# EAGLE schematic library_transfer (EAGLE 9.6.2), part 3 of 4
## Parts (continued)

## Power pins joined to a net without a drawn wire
3V3(OUT): U73.36(3V3(OUT))
3V3OUT: U181.17(3V3OUT)
ADC_AVDD: U70.43(ADC_AVDD)
AGND: U181.25(AGND)
DVDD: U70.23(DVDD) U70.50(DVDD)
EXP: U38.29(EXP)
GND: U34.1(GND) U38.15(GND) U38.23(GND) U38.26(GND) U70.57(GND) U73.3(GND) U73.8(GND) U73.13(GND) U73.18(GND) U73.23(GND) U73.28(GND) U73.33(GND) U73.38(GND) U135.16(GND) U147.1(GND)
GND1: U181.7(GND1)
GND2: U181.18(GND2)
GND3: U181.21(GND3)
GND_2: U135.1(GND_2)
GND_3: U135.6(GND_3)
GND_4: U135.8(GND_4)
GND_5: U135.9(GND_5)
IOVDD: U70.1(IOVDD) U70.10(IOVDD) U70.22(IOVDD) U70.33(IOVDD) U70.42(IOVDD) U70.49(IOVDD)
SWGND: U73.42(SWGND)
USB_VDD: U70.48(USB_VDD)
V+: U34.8(V+) U147.8(V+)
VBAT_ANA: U38.3(VBAT_ANA)
VBAT_DIG: U38.14(VBAT_DIG)
VBAT_RF: U38.24(VBAT_RF)
VBUS: U73.40(VBUS)
VCC: U115.14(VCC) U181.20(VCC)
VCCIO: U181.4(VCCIO)
VR_ANA: U38.2(VR_ANA)
VR_DIG: U38.4(VR_DIG)
VR_PA: U38.25(VR_PA)
VSYS: U73.39(VSYS)

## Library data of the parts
A1 = ruark2:SA818: NiceRF SA818 1W Embedded walkie talkie module
A2 = ruark2:RFM69HCW: RFM69HCW WIRELESS TRANSCEIVER 91; PARTNO: 1568-1394-ND
A3 = ruark2:PCN2-S: Isolated Module DC DC Converter 1 Output 12V 167mA 10.8V - 13.2V Input; PARTNO: 102-3935-ND
A4 = ruark2:DGVVII: Gan Module Foolishness
ANT1 = ruark2:W3010: 2.8dBi Chip antenna 1.575GHz - Antennas ROHS; JLCPCB: C6926293
ANT2 = ruark2:ANT-916-HETH: RF ANT 916MHZ HELICAL SLD TH
ANT3 = ruark2:ANT-433-HETH: 433MHz Alarms, ISM, Remote Control, Security Systems Helical RF Antenna 418MHz ~ 458MHz 1.9dBi Solder Through Hole; PARTNO: ANT-433-HETH-ND
B1 = ruark2:LEAF_BATTERY_PN: Nissan Leaf Battery P, M, N
B2 = ruark2:LEAF_BATTERY_NP: Nissan Leaf Battery N, M, P
B3 = ruark2:BU-2032SM-JJ-G
B4 = ruark2:BK-18650-PC4: HOLDER BATT LI-ION 2CELL 4PC PIN; PARTNO: BK-18650-PC4-ND
B5 = ruark2:BK-912: HOLDER COIN CELL 20MM SMD CR2032 2032; PARTNO: BK-912-ND
B6 = ruark2:BH-18650-B1BA002: 18650 JLCPCB
B7 = ruark2:BH-123A-A5BJ002: Battery case CR123A - Button And Strip Battery Connector ROHS; JLCPCB: C5290177
B8 = ruark2:BH-102B-5: Battery Holder (Open) AAA 2 Cell SMD (SMT) Tab; PARTNO: 2057-BH-102B-5-ND
B9 = ruark2:AN-2852-A: PCB Outline for Flanged Box: Metal, Aluminum Natural Cover Included 4.530" L x 2.560" W (115.06mm x 65.02mm) X 1.180" (29.97mm); PARTNO: 377-2364-ND
B10 = ruark2:AN-1320-A: PCB Outline for: Box Metal, Aluminum Natural Cover Included 4.040" L x 2.070" W (102.62mm x 52.58mm) X 1.000" (25.40mm); PARTNO: 377-2405-ND
B11 B12 = ruark2:18350: Ecigarette Battery
B13 = ruark2:2479: HOLDER BATTERY 3CELL AAA PC MNT; PARTNO: 36-2479-ND
B14 = ruark2:1042: Battery Holder (Open) 18650 1 Cell SMD (SMT) Tab; PARTNO: 36-1042-ND
B15 = ruark2:967: Battery Connector, Snap 9V 1 Cell PC Pin; PARTNO: 36-967-ND
B16 = ruark2:0805_BEAD: FERRITE BEAD 120 OHM 0805 1LN; PARTNO: 240-2393-1-ND
B17 = ruark2:53X2: Two 53 battery holders in AA configuration: Battery Contact Clip A, AA 1 Cell SMD (SMT) Tab; PARTNO: 36-53-ND
C1 = ruark2:KRM55TR72J474MH01K: 0.47µF ±20% 630V Ceramic Capacitor X7R SMD, J-Lead; PARTNO: 490-16845-1-ND
C2 = ruark2:UVR2A471MHD: 470µF 100V Aluminum Electrolytic Capacitors Radial, Can 2000 Hrs @ 85°C; PARTNO: 493-1151-ND
C3 = ruark2:UCL1E681MNL1GS: 680µF 25V Aluminum Electrolytic Capacitors Radial, Can - SMD 2000 Hrs @ 105°C; PARTNO: 493-3946-1-ND
C4 = ruark2:TZBXXX: 8.5 ~ 40pF Trimmer Capacitor 100V Top Surface Mount; PARTNO: 490-1978-1-ND
C5 = ruark2:T521X227M016ATE035: 220µF Molded Tantalum Polymer Capacitor 16V 2917 (7343 Metric) 35mOhm @ 100kHz; PARTNO: 399-9789-1-ND
C6 = ruark2:SLPX271M200A1P3: 270µF 200V Aluminum Electrolytic Capacitors Radial, Can - Snap-In 737 mOhm @ 120Hz 3000 Hrs @ 85°C, 22mm diameter, 25mm height; PARTNO: 338-1600-ND
C7 = ruark2:R60IR51005040K: 10µF Film Capacitor 160V 250V Polyester, Polyethylene Terephthalate (PET), Metallized Radial; PARTNO: 399-12481-ND
C8 = ruark2:R60IN4100AA30K: 1µF Film Capacitor 160V 250V Polyester, Polyethylene Terephthalate (PET), Metallized Radial
C9 = ruark2:PHE450SD5330JR06L2: 0.033µF Film Capacitor 700V 2000V (2kV) Polypropylene (PP), Metallized Radial; PARTNO: 399-7633-ND
C10 = ruark2:MEGACAP: 2.2µF ±20% 250V Ceramic Capacitor X7T Stacked SMD, 2 J-Lead; PARTNO: 445-7099-1-ND
C11 = ruark2:JZ300: 5.5 ~ 30pF Trimmer Capacitor 125V Top Surface Mount; PARTNO: 1674-1005-1-ND
C12 = ruark2:JZ030: 1.5 ~ 3pF Trimmer Capacitor 125V Top Surface Mount
C13 = ruark2:FE37M6C0206KB: 20µF Film Capacitor 900V Polypropylene (PP), Metallized Radial - 4 Leads; PARTNO: 478-7241-ND
C14 = ruark2:EMVY101ARA101MKE0S: 100µF 100V Aluminum Electrolytic Capacitors Radial, Can - SMD 5000 Hrs @ 105°C; PARTNO: 565-2511-1-ND
C15 = ruark2:EKYB630ELL102ML25S: 1000µF 63V Aluminum Electrolytic Capacitors Radial, Can 10000 Hrs @ 105°C, 2.73A; PARTNO: 565-3974-ND
C16 = ruark2:EEE-TG1E221UP: CAP ALUM 220UF 20% 25V SMD 500mOhm; PARTNO: PCE4063CT-ND
C17 = ruark2:EEE-HC1C101XP: 100µF 16V Aluminum Electrolytic Capacitors Radial, Can - SMD 3000 Hrs @ 105°C; PARTNO: PCE3750CT-ND
C18 = ruark2:C4AQSBW4600A3FJ: 6µF Film Capacitor 1500V (1.5kV) Polypropylene (PP), Metallized Radial - 4 Leads; PARTNO: 399-16963-ND
C19 = ruark2:B32529C6102K289: 1000 pF Film Capacitor 200V 400V Polyester, Polyethylene Terephthalate (PET), Metallized - Stacked Radial; PARTNO: 495-2564-1-ND
C20 = ruark2:A768MS277M1GLAV022: 270 µF 40 V Aluminum - Polymer Capacitors Radial, Can - SMD 22mOhm 2000 Hrs @ 125°C; PARTNO: 399-A768MS277M1GLAV022CT-ND
C21 = ruark2:A759TC227M2EAAE250: 220 µF 250 V Aluminum - Polymer Capacitors Radial, Can 250mOhm 2000 Hrs @ 125°C; PARTNO: 399-A759TC227M2EAAE250-ND
C22 = ruark2:06035C103KAT4A: ±10% 50V 0.01uF Ceramic Capacitor X7R 0603 (1608 Metric); PARTNO: 478-10055-1-ND
C23 = ruark2:06033C104KAT4A: ±10% 25V Ceramic Capacitor X7R 0603 (1608 Metric); PARTNO: 478-7018-1-ND
C24 = ruark2:1210_CAPACITOR: NO VALUE
C25 = ruark2:825MMR250K: 8.2µF Film Capacitor 160V 250V Polyester, Metallized Radial, 10%
C26 = ruark2:0805_CAPACITOR: NO DEFINED PN
C27 = ruark2:0603_CAPACITOR: 0603 Capacitor -- WARNING: NO DEFINED VALUE OR PART NUMBER
C28 = ruark2:0402_CAPACITOR: 0402 select capacitor
C29 = ruark2:200KXW330MEFC16X35: 330µF 200V Aluminum Electrolytic Capacitors Radial, Can 2000 Hrs @ 105°C; PARTNO: 1189-1727-ND
C30 = ruark2:100UF_100V_EEV-TG2A101M: 100µF 100V Aluminum Electrolytic Capacitors Radial, Can - SMD 300 mOhm @ 100kHz 2000 Hrs @ 125°C; PARTNO: PCE3695CT-ND
C31 = ruark2:25PK4700MEFC16X25: 4700µF 25V Aluminum Electrolytic Capacitors Radial, Can 2000 Hrs @ 85°C 0.63"; PARTNO: 1189-1732-ND
C32 = ruark2:10CMCAP: 47000µF 16V Aluminum Electrolytic Capacitor ESMH160VSN473MR50T; PARTNO: 565-2620-ND
CM1 = ruark2:RPI_CM3+
CR1 = ruark2:US1M-13-F: Diode Standard 1000V 1A 10pF 75ns Surface Mount SMA; PARTNO: US1M-FDICT-ND
CR2 = ruark2:UPP1001E3/TR7: RF Diode PIN - Single 100V 2.5W DO-216; PARTNO: UPP1001E3/TR7CT-ND
CR3 = ruark2:TSSA5U50_EG3: Diode Schottky 50V 5A Surface Mount DO-214AC (SMA); PARTNO: TSSA5U50E3GCT-ND
CR4 = ruark2:TPMR6J-S1G: Diode Standard 600V 6A Surface Mount TO-277A (SMPC); PARTNO: TPMR6JS1GCT-ND
CR5 = ruark2:STPSC20H12CWL: Diode Array 1 Pair Common Cathode Silicon Carbide Schottky 1200V 25A Through Hole TO-247-3; PARTNO: 497-17246-ND
CR6 = ruark2:STPS30SM100SG-TR: DIODE SCHOTTKY 100V 30A D2PAK; PARTNO: STPS30SM100SG-TR
CR7 CR8 = ruark2:SMP1345-040LF: RF Diode PIN - Single 50V 150mA 750mW 0402; PARTNO: 863-1145-1-ND
CR9 = ruark2:SMAJ20A: 32.4V Clamp 12.3A Ipp Tvs Diode Surface Mount DO-214AC; PARTNO: 732-SMAJ20ACT-ND
CR10 = ruark2:S1GTR: Diode Standard 400V 1A Surface Mount SMA (DO-214AC); PARTNO: 1655-1504-1-ND
CR11 = ruark2:RFN6BM2DFHTL: SUPER FAST RECOVERY DIODE 200V 6A DPAK; PARTNO: RFN6BM2DFHTLCT-ND
CR12 = ruark2:PMEG6010CEGWX: Diode Schottky 60V 1A Surface Mount SOD-123; PARTNO: 1727-7339-6-ND
CR13 = ruark2:PDS4150: Diode Schottky 150V 4A Surface Mount PowerDI™ 5; PARTNO: PDS4150DICT-ND
CR14 = ruark2:MBRB20200CTG: Diode Array 1 Pair Common Cathode Schottky 200V 10A Surface Mount TO-263-3, D²Pak (2 Leads + Tab), TO-263AB; PARTNO: MBRB20200CTGOS-ND
CR15 = ruark2:FSV20100V: Diode Schottky 100V 20A Surface Mount TO-277-3; PARTNO: FSV20100VCT-ND
CR16 = ruark2:ES1JFL: Diode Standard 600 V 1A Surface Mount SOD-123F; PARTNO: ES1JFLCT-ND
CR17 = ruark2:BZT52C10-TP: Zener Diode 10V 500mW ±6% Surface Mount SOD-123; PARTNO: BZT52C10-TPMSCT-ND
CR18 = ruark2:BAS21GWX: Diode Standard 200V 225mA (DC) Surface Mount SOD-123; PARTNO: 1727-7323-1-ND
CR19 = ruark2:BAP64-03,115: RF Diode PIN - Single 175V 100mA 500mW SOD-323; PARTNO: 568-1930-1-ND
CR20 = ruark2:824501601: 96.8V Clamp 4.1A Ipp Tvs Diode Surface Mount DO-214AC; PARTNO: 732-824501601CT-ND
CR21 = ruark2:824501401: 64.5V Clamp 6.1A Ipp Tvs Diode Surface Mount DO-214AC; PARTNO: 732-9960-1-ND
CR22 = ruark2:150060RS75000: Red 625nm LED Indication - Discrete 2V 0603 (1608 Metric); PARTNO: 732-4978-1-ND
D1 = ruark2:WP934MD/2ID: LED Circuit Board Indicator LED Circuit Board Indicator 2 High Red (x 2) Diffused, Tinted 2V 30mA Round with Domed Top 3mm, T-1 Through Hole, Right Angle. Compatible with SSF-LXH240IID
D2 = ruark2:VSSAF510-M3/H: Diode Schottky 100V 5A Surface Mount DO-221AC (SlimSMA); PARTNO: VSSAF510-M3/HGICT-ND
D3 = ruark2:VEMD5160X01: Photodiode 840nm 30ns 130° 4-TDFN Exposed Pad; PARTNO: VEMD5160X01CT-ND
D4 = ruark2:STPS20SM60D: Diode Schottky 60V 20A Through Hole TO-220AC; PARTNO: 497-12305-ND
D5 = ruark2:SS24FL: Diode Schottky 40V 2A Surface Mount SOD-123F; PARTNO: SS24FLCT-ND
D6 = ruark2:SP4022-01FTG: 35V Clamp 15A (8/20µs) Ipp Tvs Diode Surface Mount SOD-323; PARTNO: F6756CT-ND
D7 = ruark2:SP3003-02JTG: 15V Clamp 2.5A (8/20µs) Ipp Tvs Diode Surface Mount SC-70-5 JLCPCB: C151302; PARTNO: F3301CT-ND
D8 = ruark2:SMP1330-005LF: RF Diode Standard - 1 Pair Series Connection 20V 100 mA 250 mW SOT-23-3; PARTNO: 863-1101-1-ND
D9 = ruark2:SMAJ5.0CA/TR7: 9.2V Clamp 43.5A Ipp Tvs Diode Surface Mount DO-214AC (SMA)
D10 = ruark2:SM4007PL: 1A 1kV 1.1V@1A SOD-123FL Diodes - General Purpose ROHS
D11 = ruark2:SK12-SK110
D12 = ruark2:SH18101AS: eBay Gian LED 7 Segment
D13 = ruark2:SFH-2400-Z: Photodiode 900nm 5ns 120° 3-SMD, Gull Wing; PARTNO: 475-2662-1-ND
D14 = ruark2:SDUR520: Diode Standard 200V Through Hole TO-220AC; PARTNO: 1655-1191-ND
D15 = ruark2:SBRD8835LG-VF01: Diode Schottky 35V 8A Surface Mount DPAK; PARTNO: SBRD8835LG-VF01-ND
D16 = ruark2:PMEG6030EVPX: Diode Schottky 60 V 3A Surface Mount SOD-128/CFP5; PARTNO: 1727-1349-1-ND
D17 = ruark2:PDZ15BGWX: Zener Diode 15V 365mW ±2.13% Surface Mount SOD-123; PARTNO: 1727-7703-1-ND
D18 = ruark2:NSR0340HT1G: Diode 40 V 250mA Surface Mount SOD-323
D19 = ruark2:MBRM130LT1G: Diode Schottky 30V 1A Surface Mount Powermite; PARTNO: MBRM130LT1GOSCT-ND; VAUE: 30V, 1A
D20 = ruark2:LM4040: Shunt Voltage Reference 2.5V IC ±1% 15mA SOT-23; PARTNO: LM4040D25FCT-ND
D21 = ruark2:GWQ9LR33.PM-M4N3-XX56-1-180-R18: LED Lighting OSCONIQ® S 5050 White, Warm 3500K 5.52V 180mA 120° 2020 (5050 Metric); PARTNO: 475-GWQ9LR33.PM-M4N3-XX56-1-180-R18CT-ND
D22 = ruark2:FSV8100V: Diode Schottky 100V 8A Surface Mount TO-277-3; PARTNO: FSV8100VCT-ND
D23 = ruark2:ESDA25P35-1U1M: 41V Clamp 35A (8/20µs) Ipp Tvs Diode Surface Mount 1610; PARTNO: 497-16913-1-ND
D24 = ruark2:CRS01(TE85L,Q,M): Diode 30 V 1A Surface Mount S-FLAT (1.6x3.5), 360mV@1A, 40pF; PARTNO: CRS01QCT-ND
D25 = ruark2:CJ431: 2.5V~36V -25℃~+85℃@(TA) ±0.5% 1mA 100mA 50ppm/℃ Adjustable SOT-23(SOT-23-3) Voltage References ROHS
D26 = ruark2:BZX84C12LT1G: Zener Diode 12V 250mW ±5% Surface Mount SOT-23-3 (TO-236); PARTNO: BZX84C12LT1GOSCT-ND
D27 = ruark2:BPW34FS-Z: Photodiode 950nm 20ns 120° 2-SMD, Gull Wing Daylight filter; PARTNO: 475-3518-1-ND
D28 D30 = ruark2:BPW34: Photodiode 850nm 20ns 120° 2-DIP (0.213", 5.40mm); PARTNO: 475-1070-ND
D29 D31 = ruark2:BPW24_SMD: Surface Mount BPW24
D32 = ruark2:156120RS75300: Red 624nm LED Indication - Discrete 2V 1206 Reverse Mount (3216 Metric); PARTNO: 732-5031-1-ND
D33 = ruark2:15SQ045TR: Diode Schottky 45V 15A Through Hole R-6; PARTNO: 1655-1354-1-ND
D34 = ruark2:1SMA5937BT3G: Zener Diode 33 V 1.5 W ±5% Surface Mount SMA
D35 = ruark2:1PS79SB70,115: Diode Schottky 70mA (DC) Surface Mount SOD-523 70V 2pF; PARTNO: 1727-4784-1-ND
D36 = ruark2:1N4148WS: Diode 75 V 150mA Surface Mount SOD-323; PARTNO: 1N4148WS-FDICT-ND
F1-F6 = ruark2:PCB_FUSE: PCB Trace Fuse Replaceable by 1206 Fuse
F7 = ruark2:LITTLEFUSE: FUSE BRD MNT 10A 125VAC/VDC SMD; PARTNO: F1251CT-ND
F8 = ruark2:B39232B9628P810: FILTER SAW 2.35GHZ 5SMD; PARTNO: B39232B9628P810CT-ND
F9 = ruark2:03540101ZXGY: Fuse Block 15A 600V 1 Circuit Cartridge PCB; PARTNO: F1498-ND
F10 = ruark2:3522-2: FUSE CLIP BLADE 500V 20A PCB; PARTNO: 36-3522-2-ND
F11 = ruark2:03510SS-05N-AA-00: Fan Tubeaxial 5VDC Square - 35mm L x 35mm H Sleeve 5.7 CFM (0.160m³/min) 2 Wire Leads; PARTNO: 12-03510SS-05N-AA-00-ND
F12 = ruark2:3368: Fan Tubeaxial 5VDC Square - 30mm L x 30mm H 2 Position Rectangular Connector; PARTNO: 1528-1904-ND
F13-F15 = ruark2:1206_FUSE
F16 = ruark2:0PTF015BP: Fuse Holder 1 Circuit Cartridge Through Hole 5mmx20mm; PARTNO: F6245-ND
FB1 = ruark2:2518065007Y6: 1 Signal Line Ferrite Bead 1806 (4516 Metric) 6A 10mOhm; PARTNO: 1934-1466-1-ND
GDT1 = ruark2:B88069X5641T902: Gas Discharge Tube 1200V 1000A (1kA) ±15% 2 Pole Surface Mount; PARTNO: 495-76508-1-ND
GDT2 = ruark2:2093-300-SM-RPLF: Gas Discharge Tube 3000V 3000A (3kA) ±20% 2 Pole Surface Mount; PARTNO: 2093-300-SM-RPLFCT-ND
GDT3 = ruark2:2036-60-SM-RPLF: Gas Discharge Tube 600 V 10000A (10kA) ±20% 3 Pole Surface Mount LCSC Knockoff SE90-600X; PARTNO: 2036-60-SM-RPLFCT-ND
HS1 = ruark2:WAVE-35-21: Heat Sink BGA Aluminum Alloy Board Level; PARTNO: 345-1538-ND
HS2 = ruark2:CR401-75AE-ND: Heat Sink TO-401 Aluminum Alloy Board Level, Vertical; PARTNO: CR401-75AE-ND
HS3 = ruark2:ATS-FPX035035025-58-C1-R0: 35x35 heatsink Heat Sink Assorted (BGA, LGA, CPU, ASIC...) Aluminum Top Mount; PARTNO: ATS36160-ND
HS4 = ruark2:ATS-CPX060060025-132-C2-R0: Heat Sink 60x60x25mm Aluminum; PARTNO: ATS1758-ND
HS5 = ruark2:530002B02500G: Heat Sink TO-220 Aluminum 20.0W @ 60°C Board Level, Vertical; PARTNO: HS380-ND
HW1 = ruark2:738W-X2/01: BOM ONLY: Power Entry Connector Receptacle, Female Sockets NEMA 5-15R Panel Mount, Snap-In; PARTNO: Q337-ND
J1 = ruark2:YK2210403000G: 4 Circuit 0.250" (6.35mm) Barrier Block Connector Screws with Captive Plate; PARTNO: YK2210403000G-ND
J2 = ruark2:XT90
J3 = ruark2:XT60PW-M
J4 = ruark2:XT60PW-F
J5 = ruark2:XT60
J6 = ruark2:XT30PW-M
J7 = ruark2:USB4085-GF-A_ALT: USB - C USB 2.0 Receptacle Connector 16 Position Through Hole, Right Angle; PARTNO: 2073-USB4085-GF-ACT-ND
J8 = ruark2:USB4085-GF-A: USB - C USB 2.0 Receptacle Connector 16 Position Through Hole, Right Angle
J9 = ruark2:USB4085-GF-A: USB - C USB 2.0 Receptacle Connector 16 Position Through Hole, Right Angle; PARTNO: 2073-USB4085-GF-ACT-ND
J10 = ruark2:USB-A2VSW6: USB - A, 2x Stacked Receptacle Connector 8 Position Through Hole Verticle; PARTNO: ED2984-ND
J11 = ruark2:UP2-AH-1-TH: USB-A (USB TYPE-A) USB 2.0 Plug Connector 4 Position Through Hole, Right Angle; PARTNO: 102-3996-ND
J12 = ruark2:UJ2-AV-1-TH: USB-A (USB TYPE-A) USB 2.0 Receptacle Connector 4 Position Through Hole; PARTNO: 102-3995-ND
J13 = ruark2:TGF2965: Test fixture for TGF2965
J14 = ruark2:TBL009-254-03GY-2GY: 3 Position Wire to Board Terminal Block Horizontal with Board 0.100" (2.54mm) Through Hole; PARTNO: 102-TBL009-254-03GY-2GY-ND
J15 = ruark2:TBL009-254-02GY-2GY: 2 Position Wire to Board Terminal Block Horizontal with Board 0.100" (2.54mm) Through Hole; PARTNO: 102-TBL009-254-02GY-2GY-ND
J16 = ruark2:SMA_0732511150: SMA Connector Receptacle, Female Socket 50 Ohm Board Edge, End Launch Solder; PARTNO: WM5534-ND
J17 = ruark2:SMAFSTJ.B.HT: SMA Connector Jack, Female Socket 50 Ohm Board Edge, End Launch Solder; PARTNO: 931-1175-ND
J18 = ruark2:SJ2-35853A-SMT: 3.5mm TRS Jack SMD
J19 = ruark2:SJ1-3524N: 3.50mm (0.141", 1/8", Mini Plug) - Headphone Phone Jack Stereo Connector Solder; PARTNO: CP1-3524N-ND
J20 = ruark2:SJ-2523-SMT: 2.5mm TRS Jack SMD
J21 = ruark2:SJ-2509N: 2.50mm (0.094", 3/32", Sub Mini, Miniature) - Headphone Phone Jack Stereo Connector Solder; PARTNO: CP-S2509N-ND
J22 = ruark2:SJ-2504A-SMT-TR: 2.50mm (0.094", 3/32", Sub Mini, Miniature) - Headphone Phone Jack Stereo (4 Conductor, TRRS) Connector Solder; PARTNO: SJ-2504A-SMT-TR
J23 = ruark2:RENAME: Jumper part for net rename. Use discouraged
J24 = ruark2:PM20C05VBDN: CONN HEADER SMD 10POS 2MM; PARTNO: 1849-1015-ND
J25 = ruark2:PCB.SMAFSTJ.B.HT: SMA Connector Jack, Female Socket 50Ohm Surface Mount Solder; PARTNO: 931-1609-ND
J26 = ruark2:MEM2080-00-128-00-A: 9 (8 + 1) Position Card Connector Secure Digital - microSD™ Surface Mount, Right Angle Gold; PARTNO: 2073-MEM2080-00-128-00-ACT-ND
J27 = ruark2:MEM2067-02-180-00-A: Micro SD, uSD, Secure Digital Memory Card Holder; PARTNO: 2073-MEM2067-02-180-00-ACT-ND
J28 = ruark2:LD15S24A4GV00LF: 15 Position D-Sub Receptacle, Female Sockets Connector; PARTNO: 609-5195-ND
J29 = ruark2:LD09P24A4GV00LF: 9 Position Vertical D-Sub Plug, Male Pins Connector; PARTNO: 609-5184-ND
J30 = ruark2:KF141R-2.54-3P: 1 2.54mm 20~26 2A Through Hole 150V 3 Push-Pull,P=2.54mm Spring Clamp System Terminal Block ROHS
J31 = ruark2:KF141R-2.54-2P: 1 2.54mm 20~26 2A Through Hole 150V 2 Push-Pull,P=2.54mm Spring Clamp System Terminal Block ROHS; JLC: C475124
J32 = ruark2:G-1005B: Power Barrel Connector Jack 2.50mm ID (0.098"), 5.50mm OD (0.217") Through Hole, Right Angle; PARTNO: 1939-G-1005B-ND
J33 = ruark2:CONUFL001-SMD
J34 = ruark2:CON-SMA-EDGE-S: SMA Connector Jack, Female Socket Board Edge, End Launch Solder; PARTNO: CON-SMA-EDGE-S-ND
J35 = ruark2:BMIV3
J36 = ruark2:BM04B-GHS-TBT(LF)(SN)(N): JST GH Connector Header Surface Mount 4 position pin 0.049" (1.25mm); PARTNO: 455-1580-1-ND
J37 = ruark2:BANANA: JACK NON-INSULATED .218" Banana; PARTNO: 36-575-4-ND
J38 = ruark2:B5B-XH-A: JST XH Connector Header Through Hole 4 position 0.098" (2.50mm); PARTNO: 455-2249-ND
J39 = ruark2:AWHW_40G-SMD: Connector Header Surface Mount 40 position 0.100" (2.54mm); PARTNO: AE11096-ND
J40 = ruark2:AU-Y1008: USB-A (USB TYPE-A), Stacked USB 1.1 Receptacle Connector 8 Position Through Hole, Right Angle; PARTNO: AE1086-ND
J41 = ruark2:AU-Y1006: USB - A USB 1.1 Receptacle Connector 4 Position Surface Mount, Right Angle; PARTNO: AE11182-ND
J42 = ruark2:ARJ-169: 1 Port RJ45 with USB A Magjack Connector Through Hole 10/100 Base-T; PARTNO: 535-13147-ND
J43 = ruark2:AFC01-S24FCA-00: OV2640 Connector Clamshell 24P Bottom Contact Surface Mount，Right Angle 0.5mm SMD,P=0.5mm,Surface Mount，Right Angle FFC/FPC Connectors ROHS; JLCPCB: C262669
J44 J76 = ruark2:16008-83-4810: Pin Receptacle Connector 0.078" ~ 0.096" (1.98mm ~ 2.44mm) No Tail Solder tip; PARTNO: 1212-16008-83-4810-ND
J45 = ruark2:A-DS09A/KG-T4S: DB9 9 Position D-Sub Plug, Male Pins Connector; PARTNO: AE10970-ND
J46 = ruark2:A-DS09A/KG-T2S: 9 Position D-Sub Plug, Male Pins Connector; PARTNO: AE10968-ND
J47 = ruark2:A-2004-2-4-LPS-N-R: Jack Modular Connector 8p8c (RJ45, Ethernet) 90° Angle (Right) Shielded Asian alternate: RCH RC00994; PARTNO: AE10387-ND
J48 = ruark2:9774100151R: Round Standoff Threaded M2.5x0.45 Steel 0.394" (10.00mm); PARTNO: 732-7117-1-ND
J49 = ruark2:691411410002: 2 Position Wire to Board Terminal Block Horizontal with Board 0.300" (7.62mm) Through Hole; PARTNO: 732-11084-ND
J50 = ruark2:691305140002: TERM BLOCK HEADER 2POS 90 3.5MM; PARTNO: 732-11063-ND
J51 = ruark2:0878980524: 5 Positions Header, Breakaway Connector 0.100" (2.54mm) Surface Mount Gold; PARTNO: WM14825-ND
J52 = ruark2:0733910070: SMA Connector Receptacle, Female Socket 50Ohm Through Hole Solder; PARTNO: WM5544-ND
J53 = ruark2:0731711900: BNC Connector Jack, Female Socket 75Ohm Through Hole Solder; PARTNO: WM5517-ND
J54 = ruark2:0731385033: BNC Connector Jack, Female Socket 50Ohm Panel Mount, Through Hole, Right Angle Solder; PARTNO: WM5515-ND
J55 = ruark2:0705430001: Connector Header Through Hole 2 position 0.100" (2.54mm); PARTNO: WM4800-ND
J56 = ruark2:0541044031: CONN FFC TOP 40POS 0.50MM R/A; PARTNO: WM3431CT-ND
J57 = ruark2:0530480210: Connector Header Through Hole, Right Angle 2 position 0.049" (1.25mm); PARTNO: WM1742-ND
J58 = ruark2:0526100872: 8 Position FPC Connector Contacts, Vertical - 1 Sided 0.039" (1.00mm) Surface Mount; PARTNO: WM6761CT-ND
J59 = ruark2:0395443002: 2 Position Wire to Board Terminal Block Horizontal with Board 0.200" (5.08mm) Through Hole; PARTNO: WM7853-ND
J60 = ruark2:0026604030: Connector Header Through Hole 3 position 0.156" (3.96mm); PARTNO: WM4621-ND
J61 = ruark2:0015913034: Molex SL 3 Positions Header Connector 0.100" (2.54mm) Surface Mount, Right Angle Tin; PARTNO: WM1376-ND
J62 = ruark2:10104110-0001LF: USB - micro B USB 2.0 Receptacle Connector 5 Position Surface Mount, Right Angle; PARTNO: 609-4052-1-ND
J63 = ruark2:10053363-200LF: 64 (Power) Position Female Connector Non Specified - Dual Edge Gold 0.100" (2.54mm) Black; PARTNO: 609-2861-ND
J64 = ruark2:10033526-N3212LF: USB - mini B Receptacle Connector 5 Position Surface Mount, Right Angle; PARTNO: 609-4700-1-ND
J65 = ruark2:5555153-1: Jack Modular Connector 8p8c (RJ45, Ethernet) 90° Angle (Right) Shielded Cat3; PARTNO: A31438-ND
J66 = ruark2:5413631-1: BNC Connector Jack, Female Socket 50 Ohm Through Hole, Right Angle Solder; PARTNO: A32270-ND
J67 = ruark2:1778625: 2 Position Terminal Block Header, Male Pins, Shrouded (4 Side) 0.098" (2.50mm) 90°, Right Angle Through Hole; PARTNO: 277-2308-1-ND
J68 = ruark2:1702473: 2 Position Wire to Board Terminal Block Horizontal with Board 0.098" (2.50mm) Surface Mount; PARTNO: 277-2337-1-ND
J69 = ruark2:01010002Z: SMD Fuse Clip 15 A 250V 1 Circuit Cartridge Chassis Mount; PARTNO: F4080-ND
J70 = ruark2:54601-906001WPLF: Jack Modular Connector 6p2c (RJ11) 90° Angle (Right) Unshielded Cat3; PARTNO: 609-5354-ND
J71 = ruark2:54202-G08-03: Connector Header Surface Mount 6 position 0.100" (2.54mm); PARTNO: 609-5602-ND
J72 = ruark2:43045-0800: Connector Header Through Hole, Right Angle 8 position 0.118" (3.00mm); PARTNO: WM1816-ND
J73 = ruark2:43045-0600: Connector Header Through Hole, Right Angle 6 position 0.118" (3.00mm); PARTNO: WM1815-ND
J74 = ruark2:43045-0400: Connector Header Through Hole, Right Angle 4 position 0.118" (3.00mm); PARTNO: WM1814-ND
J75 = ruark2:43045-0200: 2 Positions Header Connector Through Hole, Right Angle Tin; PARTNO: WM1813-ND
J77 = ruark2:9837-0-15-80-14-27-10-0: Pin Receptacle Connector 0.065" ~ 0.082" (1.65mm ~ 2.08mm) No Tail Solder; PARTNO: ED10170-ND
J78 = ruark2:8190: 4 Pin Screw Terminal, Power Tap 6-32 Through Hole, Right Angle; PARTNO: 36-8190-ND
J79 = ruark2:7792: 4 Pin Screw Terminal, Power Tap M4 Through Hole, Right Angle
J80 = ruark2:4300.0101: Power Entry Connector Receptacle, Male Pins IEC 320-C6 Panel Mount, Flange; Through Hole, Right Angle; PARTNO: 486-2099-ND
J81 = ruark2:3221-14-0300-00: Connector Header Surface Mount 14 position 0.050" (1.27mm)
J82 = ruark2:2001-1-2-21-00-BK: HDMI - Mini Receptacle Connector 19 Position Surface Mount, Right Angle; Through Hole; PARTNO: 1175-1704-1-ND
J83 = ruark2:572-0100: Test Jack, 10 A, 1.8 mm, 250 Vrms, Black, 572 Series; PARTNO: 45M6897
J84 = ruark2:24.243.1: 24.243.1 is a 4mm red test socket with silver plated brass body and ABS insulation. This socket can be mounted on PCB. Banana da da da da da; MANUFACTURER_PART_NUMBER: 24.243.1; MFR_NAME: Multicomp
J85 = ruark2:3-1470209-3: 20 Position Receptacle Connector 0.079" (2.00mm) Through Hole Gold; PARTNO: 3-1470209-3-ND
J86 = ruark2:2PINANDERSON
J87 = ruark2:2PH2-10-UA: Connector Header Through Hole 10 position 0.079" (2.00mm); PARTNO: 2057-2PH2-10-UA-ND
J88 = ruark2:1-2314820-0: 10 Position Receptacle Connector 0.079" (2.00mm) Through Hole Gold; PARTNO: 17-1-2314820-0-ND
L1 = ruark2:XAL8080-223MED: 22uH 33mOhm 5.9A Inductor
L2 = ruark2:XAL7070-473MEC: 47 µH Shielded Inductor 4.1 A 97.07mOhm Max Nonstandard
L3 = ruark2:XAL6060-223MEC: Fixed Inductors 22uH Shld 20% 5A 60.63mOhms AECQ2
L4 = ruark2:XAL4030-332: Fixed Inductors 3.3uH 20% 6.6A 28.6mOhms AEC-Q200; PARTNO: 994-XAL4030-332MEC
L5 = ruark2:TMPC0603H-220MG-D: 2A 22uH ±20% SMD Power Inductors ROHS
L6 = ruark2:TMPC0603H-100MG-D: 3.5A 10uH ±20% SMD Power Inductors ROHS
L7 = ruark2:TMPC0603H-1R0MG-D: 11A 1uH ±20% SMD Power Inductors ROHS
L8 = ruark2:SSL1306T-180M-N: 3.7A 18uH ±20% 7.5A SMD Power Inductors ROHS JLCPCB: C329890
L9 = ruark2:SRR1210-470M: 47 µH Shielded Drum Core, Wirewound Inductor 3.8 A 72mOhm Max Nonstandard; PARTNO: SRR1210-470MCT-ND
L10 = ruark2:SRR1208-270ML: 27µH Shielded Wirewound Inductor 3A 48 mOhm Max Nonstandard; PARTNO: SRR1208-270MLCT-ND
L11 = ruark2:SRR1208-6R5ML: FIXED IND 6.5UH 6A 18 MOHM SMD; PARTNO: SRR1208-6R5MLCT-ND
L12 = ruark2:SRP1265C-100M: 10µH Shielded Wirewound Inductor 12A 18mOhm Max Nonstandard; PARTNO: SRP1265A-220MCT-ND
L13 = ruark2:SRP1265A-220M: 22µH Shielded Wirewound Inductor 9A 37mOhm Max Nonstandard; PARTNO: SRP1265A-220MCT-ND
L14 = ruark2:SRN8040TA-R50Y: 500 nH Semi-Shielded Drum Core, Wirewound Inductor 12 A 5.5mOhm Nonstandard; PARTNO: SRN8040TA-R50YCT-ND
L15 = ruark2:SRN8040TA-1R0Y: FIXED IND 1UH 8.5A 8.2 MOHM SMD; PARTNO: SRN8040TA-1R0YCT-ND
L16 = ruark2:SNR5040TYD102M: 1mH ±20% SMD Power Inductors ROHS 200mA; JLCPCB: C2827402
L17 = ruark2:SMCM090605-102: 1000uH@100kHz 6kΩ@10MHz 0.31Ω 2 SMD,9.0x6.0x5.0mm Common Mode Filters ROHS
L18 = ruark2:SDR1005-103KL: 10 mH Unshielded Wirewound Inductor 100 mA 39Ohm Max Nonstandard 100mA; PARTNO: SDR1005-103KLCT-ND
L19 = ruark2:SDR0603-391KL: 390µH Unshielded Wirewound Inductor 180mA 3.4 Ohm Max Nonstandard; PARTNO: SDR0603-391KLCT-ND
L20 = ruark2:SDR0403-330KL: 33 µH Unshielded Drum Core, Wirewound Inductor 640 mA 540mOhm Max Nonstandard; PARTNO: SDR0403-330KLCT-ND
L21 = ruark2:SDCW2520S-2-601TF: 600Ω@100MHz 0.38Ω 2 1008 Common Mode Filters ROHS JLCPCB: C843574
L22 = ruark2:PQ2614BHA-6R8K_INDUCTOR: 6.8µH Shielded Wirewound Inductor 30A 1.9 mOhm Max Nonstandard; PARTNO: PQ2614BHA-6R8K-ND
L23 = ruark2:PM2120-102K-RC: 1mH Unshielded Toroidal Inductor 2.5A 215 mOhm Max Nonstandard; PARTNO: M8801-ND
L24 = ruark2:PE-65535NL: 20mH Isolation and Data Interface (Encapsulated) Pulse Transformer 1:2CT Through Hole XFRMR 64KBPS 1:2CT 20MH T/H; PARTNO: 553-1579-5-ND
L25 = ruark2:PA0489LNL: 2.24µH Unshielded Toroidal Inductor 19A 2.7 mOhm Max Radial; PARTNO: 553-1507-ND
L26 = ruark2:NS10165T3R3NNA: 3.3µH Shielded Wirewound Inductor 6.76A 10.8 mOhm Max Nonstandard; PARTNO: 587-3149-1-ND
L27 = ruark2:NRS8030T1R5NJGJ: 1.5 µH Shielded Drum Core, Wirewound Inductor 5.3 A 15.6mOhm Max Nonstandard; PARTNO: 587-2963-1-ND
L28 = ruark2:NRS8030T1R0NJGJ: 1µH Shielded Wirewound Inductor 6.2A 11.7mOhm Max Nonstandard; PARTNO: 587-2962-1-ND
L29 = ruark2:NR6028T101M: 100 µH Shielded Wirewound Inductor 660 mA 780mOhm Max Nonstandard (Many values available in series); PARTNO: 587-2105-1-ND
L30 = ruark2:NR6028T2R2N: 2.2 µH Shielded Drum Core, Wirewound Inductor 3.7 A 26mOhm Max Nonstandard (Many values available in series); PARTNO: 587-2098-1-ND
L31 = ruark2:NR6028: 10µH Shielded Wirewound Inductor 1.9A 84.5 mOhm Max Nonstandard (Many values available in series); PARTNO: 587-2102-1-ND
L32 = ruark2:NR6020T6R8N: 6.8 µH Shielded Drum Core, Wirewound Inductor 1.8 A 102mOhm Max Nonstandard (Many values available in series); PARTNO: 587-2629-1-ND
L33 = ruark2:MSRH104R-471MT: 470uH ±20% SMD Power Inductors ROHS; JLCPCB: C915333
L34 = ruark2:LHL08TB100K: 10µH Unshielded Inductor 2.4A 41 mOhm Max Radial; PARTNO: 587-5885-1-ND
L35 = ruark2:IHLP2020CZER3R3M11: 3.3µH Shielded Molded Inductor 5.5A 40.4mOhm Max Nonstandard; PARTNO: 541-1237-6-ND
L36 = ruark2:HCTI-1000-2.4: 1mH Shielded Toroidal Inductor 2.4A 300 mOhm Max Radial; PARTNO: 595-1740-ND
L37 = ruark2:HCM1307-3R3-R: 3.3µH Shielded Inductor 15A 4.5mOhm Max Nonstandard; PARTNO: 283-4636-1-ND
L38 = ruark2:GA3092-AL: RF Inductors - SMD 3.7 nH Unshld 5% 7A 2mOhms
L39 = ruark2:FWP201610P-R33ML: 4.1A 0.33uH ±20% Molding Choke 0806 Power Inductors ROHS
L40 = ruark2:FNR8065S103MT: 130mA 10mH ±20% 22.8Ω SMD Power Inductors ROHS
L41 = ruark2:CM3421Y600R-10: 2 Line Common Mode Choke Surface Mount 60 Ohms @ 100 MHz 15A DCR 0.75mOhm; PARTNO: 240-2501-1-ND
L42 = ruark2:BRC2012T4R7MD: 4.7µH Unshielded Wirewound Inductor 600mA 344.5 mOhm Max 0805; PARTNO: 587-2907-1-ND
L43 = ruark2:B82477D4683M900: Shielded 2 Coil Inductor Array 272 µH Inductance - Connected in Series 68 µH Inductance - Connected in Parallel 107.5mOhm Max DC Resistance (DCR) - Parallel Nonstandard; PARTNO: 495-B82477D4683M900CT-ND
L44 = ruark2:ASPI-1367-100M-T: 10µH Shielded Wirewound Inductor 10A 18.5 mOhm Max Nonstandard; PARTNO: ASPI-1367-100M-TCT-ND
L45 = ruark2:APW12A10: 22uH ±20% 4.95A SMD Power Inductors ROHS JLCPCB: C311499
L46 = ruark2:ACP3225-501-2P-T000: 2 Line Common Mode Choke Surface Mount 500 Ohms @ 100 MHz 2A DCR 40mOhm (Typ); PARTNO: 445-172408-1-ND
L47 = ruark2:74438357010: FIXED IND 1UH 7.4A 13.5 MOHM SMD; PARTNO: 732-11197-1-ND
L48 = ruark2:7443634700: FIXED IND 47UH 12A 12.2 MOHM SMD; PARTNO: 732-2525-1-ND
L49 = ruark2:744272251: 250 µH @ 100 kHz 2 Line Common Mode Choke Surface Mount 970 Ohms @ 15 MHz 2A DCR 35mOhm; PARTNO: 732-1491-1-ND
L50 = ruark2:744272221: 220µH @ 100kHz 2 Line Common Mode Choke Surface Mount 780 Ohms @ 15MHz 2.2A DCR 32mOhm; PARTNO: 732-1490-1-ND
L51 = ruark2:2222SQ-111: RF Inductors - SMD 2222 110nH Unshld 2% 5.7A 6.5mOhms
L52 = ruark2:1111SQ-47N: RF Inductors - SMD 1111 47nH Unshld 2% 4.4A 11.3mOhms
L53 = ruark2:1111SQ-36NGEC: RF Inductors - SMD 1111 36nH Unshld 2% 4.8A 9.8mOhms
L54 = ruark2:0908SQ--17NGLC: Coilcraft RF Inductor 16.6nH, 5.2%, Q=130, SRF=3.7GHz, DCR=9m, Irms=4.4A
L55 = ruark2:0906--3JLC: Coilcraft RF Inductor 2.55nH, 5%, Q=100, SRF=8.2GHz, DCR=5m, Irms=1.6A
L56 = ruark2:0906--2KLC: Coilcraft Inductor 1.65nH, 10%, Q=100, SRF=1-GHz, DCR=4m, Irms=1.6A
L57 = ruark2:0806SQ--5N5GLC: Coilcraft RF Inductor 5.5nH, 2%, Q=60, SRF=4.9GHz, DCR=3.4m, Irms=2.9A
L58 = ruark2:0805INDUCTOR
L59 = ruark2:0603_INDUCTOR: 0603 Inductor: WARNING: NO DEFINED PART NUMBER OR VALUE
L60 = ruark2:0402_INDUCTOR: select
L61 = ruark2:60B473C: 47µH Unshielded Wirewound Inductor 10.5A 13 mOhm Max Nonstandard, WARNING: Murata; PARTNO: 811-2459-ND
L62 = ruark2:60A193C: 19.4µH Unshielded Wirewound Inductor 8.5A 11mOhm Max Nonstandard; PARTNO: 811-2452-1-ND
LP1 = ruark2:VLP-650-R: Light Pipe Single Clear Rigid Board Mount, Press Fit; PARTNO: 492-2537-ND
LP2 = ruark2:5151071F: Light Pipe 2 Wide Clear Rigid Round with Flat Top, 3mm Board Mount, Press Fit; PARTNO: 350-1590-ND
LP3 = ruark2:5151069F: Light Pipe 3 Wide Clear Rigid Board Mount, Press Fit, Right Angle; PARTNO: 350-2182-ND
LS1 = ruark2:PKM13EPYH4000-A0: Buzzers Transducer, Externally Driven Piezo 1.5V 4kHz 70dB @ 1.5V, 10cm Through Hole PC Pins; PARTNO: 490-4698-ND
M1 = ruark2:634: Mounting Bracket Short L 0.140" (3.56mm), 6-32 Brass, Nickel Plated; PARTNO: 36-634-ND
M2 = ruark2:40X40HS: Dumy footprint for 40x40mm heatsink
MOV1 = ruark2:MOV-07D471K: 470V 1.2kA Varistor 1 Circuit Through Hole Disc 7mm; PARTNO: MOV-07D471K-ND
Q1 = ruark2:ZXTN4004KTC: Bipolar (BJT) Transistor NPN 150V 1A 3.8W Surface Mount TO-252; PARTNO: ZXTN4004KTCDICT-ND
Q2 = ruark2:TPH3212PS: N-Channel GaN 650V 27A (Tc) 104W (Tc) Through Hole TO-220AB WARNING: Gate-Source-Drain; PARTNO: TPH3212PS-ND
Q3 = ruark2:SUP90330E: MOSFET N-CH 200V 37.5mOhm 21nC 35.8A TO220AB; PARTNO: SUP90330E-GE3-ND
Q4 = ruark2:STS11N3LLH5: N-Channel 30V 11A (Tc) 2.7W (Tc) Surface Mount 8-SO; PARTNO: 497-10310-1-ND
Q5 = ruark2:STN4NF20L: N-Channel 200V 1A (Tc) 3.3W (Tc) Surface Mount SOT-223; PARTNO: 497-10779-1-ND
Q6 = ruark2:SIS413DN-T1-GE3: P-Channel 30V 18A (Tc) 3.7W (Ta), 52W (Tc) Surface Mount PowerPAK® 1212-8; PARTNO: SIS413DN-T1-GE3CT-ND
Q7 = ruark2:SIS128LDN-T1-GE3: N-Channel 80V 10.2A (Ta), 33.7A (Tc) 3.6W (Ta), 39W (Tc) Surface Mount PowerPAK® 1212-8; PARTNO: SIS128LDN-T1-GE3CT-ND
Q8 = ruark2:SI7115DN-T1-GE3: P-Channel 150 V 8.9A (Tc) 3.7W (Ta), 52W (Tc) Surface Mount PowerPAK® 1212-8; PARTNO: SI7115DN-T1-GE3CT-ND
Q9 = ruark2:QUARTER: Outline of US Quarter for Scale
Q10 = ruark2:PSMN3R3-80BS: N-Channel 80V 120A (Tc) 306W (Tc) Surface Mount D2PAK; PARTNO: 1727-7108-1-ND
Q11 = ruark2:PMXB56EN: N-Channel 30V 3.2A (Ta) 400mW (Ta), 8.33W (Tc) Surface Mount DFN1010D-3; PARTNO: 1727-2313-1-ND
Q12 = ruark2:PMBTA45,215: Bipolar (BJT) Transistor NPN 500 V 150 mA 35MHz 300 mW Surface Mount TO-236AB; PARTNO: 1727-5332-1-ND
Q13 = ruark2:PMBTA06,235: Bipolar (BJT) Transistor NPN 80 V 500 mA 100MHz 250 mW Surface Mount TO-236AB; PARTNO: 1727-2161-1-ND
Q14 = ruark2:PHB33NQ20T,118: N-Channel 200V 32.7A (Tc) 230W (Tc) Surface Mount D2PAK, 77mOhm, 33nC; PARTNO: 1727-4765-1-ND
Q15 = ruark2:PBHV9115T,215: Bipolar (BJT) Transistor PNP 150 V 1 A 115MHz 300 mW Surface Mount TO-236AB; PARNO: 1727-5683-1-ND
Q16 = ruark2:MMBT3906-7-F: Bipolar (BJT) Transistor PNP 40V 200mA 250MHz 300mW Surface Mount SOT-23-3 (SMD 2N3906)
Q17 = ruark2:MMBT3904-TP: Bipolar (BJT) Transistor NPN 40V 200mA 300MHz 350mW Surface Mount SOT-23 (SMD 2N3904)
Q18 = ruark2:IRLR8726TRPBF: N-Channel 30V 86A (Tc) 75W (Tc) 5.8mR 23nC Surface Mount D-Pak; PARTNO: IRLR8726TRPBFCT-ND
Q19 = ruark2:IRFR8314TRPBF: N-Channel 30V 2.2mOhm 90A (Tc) 125W (Tc) Surface Mount D-PAK (TO-252AA); PARTNO: IRFR8314TRPBFCT-ND
Q20 = ruark2:IPW60R180C7XKSA1-ND: N-Channel 600V 13A (Tc) 68W (Tc) Through Hole PG-TO247-3; PARTNO: IPW60R180C7XKSA1-ND
Q21 = ruark2:IPP65R125C7XKSA1: N-Channel 650V 18A (Tc) 101W (Tc) Through Hole PG-TO-220-3; PARTNO: IPP65R125C7XKSA1-ND
Q22 = ruark2:IPB60R060P7ATMA1: N-Channel 650V 48A (Tc) 164W (Tc) Surface Mount D²PAK (TO-263AB); PARTNO: IPB60R060P7ATMA1CT-ND
Q23 = ruark2:IPA60R080P7XKSA1: N-Channel 600V 37A (Tc) 29W (Tc) Through Hole PG-TO220 Full Pack; PARTNO: IPA60R080P7XKSA1-ND
Q24 = ruark2:FQD7N10LTM: MOSFET N-CH 100V 5.8A 350mOhm 6nC DPAK; PARTNO: FQD7N10LTMCT-ND
Q25 = ruark2:FDMT800100DC: N-Channel 100 V 24A (Ta), 162A (Tc) 3.2W (Ta), 156W (Tc) Surface Mount 8-Dual Cool™88; PARTNO: FDMT800100DCCT-ND
Q26 = ruark2:FDMS8620: N-Channel 120V 13.5A (Ta) 2.7W (Ta), 156W (Tc) Surface Mount Power56; PARTNO: FDMS86202CT-ND
Q27 = ruark2:FDMC8321L: N-Channel 40 V 22A (Ta), 49A (Tc) 2.3W (Ta), 40W (Tc) Surface Mount Power33; PARTNO: FDMC8321LCT-ND
Q28 = ruark2:FDG6301N: Mosfet Array 2 N-Channel (Dual) 25V 220mA 300mW Surface Mount SC-88 (SC-70-6); PARTNO: FDG6301NCT-ND
Q29 = ruark2:EPC2021: TRANS GAN 80V 90A BUMPED DIE; PARTNO: 917-1089-1-ND
Q30 = ruark2:DMN3023L-7: N-Channel 30V 6.2A (Ta) 900mW (Ta) Surface Mount SOT-23; PARTNO: DMN3023L-7DICT-ND
Q31 = ruark2:DMN61D9UWQ-7: N-Channel 400mA (Ta) 440mW (Ta) Surface Mount SOT-323; PARTNO: DMN61D9UWQ-7-ND
Q32 = ruark2:CSD87350Q5D: Mosfet Array 2 N-Channel (Dual) 30V 40A 12W Surface Mount 8-LSON (5x6); PARTNO: 296-28318-1-ND
Q33 = ruark2:CSD16321Q5: N-Channel 25V 31A (Ta), 100A (Tc) 3.1W (Ta) Surface Mount 8-VSON-CLIP (5x6); PARTNO: 296-24517-1-ND
Q34 = ruark2:CSD16301Q2: N-Channel 25V 5A (Tc) 2.3W (Ta) Surface Mount 6-SON; PARTNO: 296-25260-1-ND
Q35 = ruark2:BUK9875-100A/CUX: MOSFET N-CH 100V 7A SOT223; PARTNO: 1727-2228-1-ND
Q36 = ruark2:BUK7660-100A,118: N-Channel 100 V 26A (Tc) 106W (Tc) Surface Mount D2PAK; PARTNO: 1727-7172-1-ND
Q37 = ruark2:BSS806NEH6327XTSA1: N-Channel 20 V 2.3A (Ta) 500mW (Ta) Surface Mount PG-SOT23; PARTNO: BSS806NEH6327XTSA1CT-ND
Q38 = ruark2:BSS138DWQ-7: Mosfet Array 2 N-Channel (Dual) 50V 200mA 200mW Surface Mount SOT-363; PARTNO: BSS138DWQ-7DICT-ND
Q39 = ruark2:AO4576: N-Channel 30V 20A (Ta) 3.1W (Ta) 9.8mOhm @ 4.5Vgs, 5.8mOhm @ 10Vgs Surface Mount 8-SOIC; PARTNO: 785-1465-1-ND
Q40 = ruark2:AO3400A: N-Channel 5.7A (Ta) 1.4W (Ta) Surface Mount SOT-23-3L
Q41 = ruark2:AFT09MS007N: RF Mosfet LDMOS 7.5V 100mA 870MHz 15.2dB 7.3W PLD-1.5W-2; PARTNO: AFT09MS007NT1CT-ND
Q42 = ruark2:AFT05MS031GNR1
Q43 = ruark2:AFT05MS003N: RF Mosfet LDMOS 7.5V 100mA 520MHz 20.8dB 3W SOT-89-3; PARTNO: AFT05MS003NT1CT-ND
R1 = ruark2:WSL2816: Vishay WSL2816 4m-100m
R2 = ruark2:ST-4ETB101: ±20% ±100ppm/℃ 250mW 100Ω SMD Variable Resistors/Potentiometers ROHS; JLCPCB: C2922093
R3 = ruark2:ST-4ETA502: 5 kOhms 0.25W, 1/4W J Lead Surface Mount Trimmer Potentiometer Cermet 1.0 Turn Top Adjustment; PARTNO: 563-ST4ETA502DKR-ND
R4 = ruark2:PTV09A-4025F-A103: 10k Ohm 1 Gang Logarithmic Through Hole, Snap In Potentiometer None 1 Turn Carbon 0.05W, 1/20W PC Pins, Board Locks; PARTNO: PTV09A-4025F-A103-ND
R5 = ruark2:PTV09A-4020F-B102: 1k Ohm 1 Gang Linear Through Hole, Snap In Potentiometer None 1 Turn Carbon 0.05W, 1/20W PC Pins, Board Locks; PARTNO: PTV09A-4020F-B102-ND
R6 = ruark2:PTV09A-4020F-A504: 500k Ohm 1 Gang Logarithmic Through Hole, Snap In Potentiometer None 1 Turn Carbon 0.05W, 1/20W PC Pins, Board Locks; PARTNO: PTV09A-4020F-A504-ND
R7 = ruark2:PTV09A-2020F-B103: 10k Ohm 1 Gang Linear Through Hole, Snap In Potentiometer None 1.0 Kierros Carbon 0.05W, 1/20W PC Pins, Board Locks; PARTNO: PTV09A-2020F-B103-ND
R8 = ruark2:P160KN
R9 = ruark2:P091S-FC20BR10K: 10k Ohm 1 Gang Linear Panel Mount Potentiometer Rotary, SPST 1.0 Kierros Conductive Plastic 0.05W, 1/20W PC Pins, Board Locks; PARTNO: 987-1283-ND
R10 = ruark2:MHR0317SA108F70: 1 GOhms ±1% 0.8W Through Hole Resistor Radial High Voltage Thick Film; PARTNO: 490-18223-ND
R11 = ruark2:3361P-1-100GLF: 10 Ohms 0.5W, 1/2W Gull Wing Surface Mount Trimmer Potentiometer Cermet 1.0 Turn Top Adjustment; PARTNO: 3361P-1-100GLFCT-ND
R12 = ruark2:2512_RESISTOR: SELECT RESISTOR; PARTNO: na
R13 = ruark2:0805_RESISTOR: NO DEFINED PN
R14 = ruark2:0603_RESISTOR: 0603 Resistor -- WARNING: NO DEFINED PART NUMBER OR VALUE
R15 = ruark2:0402_RESISTOR: 0402 Resistor -- WARNING: NO DEFINED PART NUMBER OR VALUE
RT1 = ruark2:B57330V2103J260: THERMISTOR NTC 10KOHM 3380K 0603; PARTNO: 495-5817-1-ND
S1 = ruark2:SCTLOGO: Solar Car Silkscreen Logo
S2 = ruark2:ARE10A4H: RELAY RF SPDT 500MA 4.5V; PARTNO: 255-5312-1-ND
S3 = ruark2:2118730-2_SHIELD: RF Shield Frame 1.201" (30.50mm) X 1.732" (44.00mm) Surface Mount; PARTNO: A126159CT-ND
SH1 = ruark2:2118714-2: RF Shield Frame 0.500" (12.70mm) X 0.538" (13.66mm) Surface Mount; PARTNO: A126151CT-ND
SM1 = ruark2:28BYJ-48: Mechanical footprint for 28BYJ-48 Steper motor
SW1 = ruark2:RM104772BCB: Rotary Switch 4 Position SP4T 500mA (DC) 24VDC Through Hole; PARTNO: CKN10699-ND
SW2 = ruark2:PEC12R-2220F-S0024: ENCODER ROTARY, 24 pulses per rotation, detent, mom switch; PARTNO: PEC12R-2220F-S0024-ND
SW3 = ruark2:EVQ-PF008K: Tactile Switch SPST-NO Side Actuated Through Hole, Right Angle; PARTNO: P10880S-ND
SW4 = ruark2:ESE-18LF01: Switch SPST-NO Surface Mount, Right Angle; PARTNO: P13361SCT-ND
SW5 = ruark2:A20503RSCQE: Rotary Switch 5 Position DP5T 2.5A (AC), 350mA (DC) 125 VAC Panel Mount, Through Hole; PARTNO: CKN11321-ND
SW6 = ruark2:100SP4T2B4M6RE: SWITCH TOGGLE SPDT 0.4VA 20V MOM-OFF-MOM; PARTNO: EG2391-ND
SW7 = ruark2:100SP1T2B4M6QE: Toggle Switch SPDT Through Hole, Right Angle 5A 120V; PARTNO: EG2362-ND
SW8 = ruark2:100SP1T1B4M6RE: Toggle Switch SPDT Through Hole, Right Angle; PARTNO: EG2356-ND
SW9 = ruark2:100SP1T1B1M1QEH: Toggle Switch SPDT Panel Mount; PARTNO: EG2350-ND
SW10 = ruark2:100DP1T1B1M2QEH: SWITCH TOGGLE DPDT 5A 120V; PARTNO: EG2400-ND
T1 = ruark2:TEST_POINT: Test Point
T2 = ruark2:SBM-20: SBM-20 Part Outline. Does not include connectors (fuse clips)
T3 = ruark2:MABA-010247-2R1250: RF Balun 1MHz ~ 1.6GHz 1:2 6-SMD (5 Leads), Flat Lead; PARTNO: 1465-MABA-010247-2R1250CT-ND
T4 = ruark2:H1102NLT
T5 = ruark2:ALT4532M-201-T001: 200µH LAN Pulse Transformer 1CT:1CT Surface Mount JLCPCB: C2845101; PARTNO: 445-15085-1-ND
T6 = ruark2:ACM9070-701-2PL-TL01: 2 Line Common Mode Choke Surface Mount 700 Ohms @ 100MHz 5A DCR 10mOhm; PARTNO: 445-2216-1-ND
T7 = ruark2:0399700102: 2 Position Wire to Board Terminal Block Horizontal with Board 0.400" (10.16mm) Through Hole 60A, 600V, 6AWG; DESCRIPTION: 2 Pos Term; PARTNO: 0399700102
T8 = ruark2:78615/9JC: 10mH General Purpose Pulse Transformer 1CT:1CT Surface Mount 56Vus; PARTNO: 811-2423-ND
T9 = ruark2:78615/9C: 10mH General Purpose Pulse Transformer 1CT:1CT Surface Mount 56Vus
TP1 = ruark2:5011: Black PC Test Point, Multipurpose Phosphor Bronze, Silver Plating 0.063" (1.60mm) Hole Diameter Mounting Type; PARTNO: 36-5011-ND
TP2 = ruark2:5010: Red PC Test Point, Multipurpose Phosphor Bronze, Silver Plating 0.063" (1.60mm) Hole Diameter Mounting Type; PARTNO: 36-5010-ND
TP3 = ruark2:5002: White PC Test Point, Miniature Phosphor Bronze, Silver Plating 0.040" (1.02mm) Hole Diameter Mounting Type; PARTNO: 36-5002-ND
TP4 = ruark2:5001: Black PC Test Point, Miniature Phosphor Bronze, Silver Plating 0.040" (1.02mm) Hole Diameter Mounting Type; PARTNO: 36-5001-ND
U1 = ruark2:ZXGD3003E6TA: Low-Side Gate Driver IC Non-Inverting SOT-23-6 5A; PARTNO: ZXGD3003E6CT-ND
U2 = ruark2:XC6206P332MR-G: 200mA Fixed 3.3V Positive electrode 6V SOT-23-3L Voltage Regulators - Linear, Low Drop Out (LDO) Regulators ROHS; JLC: C5446
U3 = ruark2:XC6206-2.8V: 250mA Fixed 2.8V Positive electrode 6V SOT-23-3L Linear Voltage Regulators (LDO) ROHS
U4 = ruark2:XBP9X-DMRS-001: General ISM under 1GHz Transceiver Module 902MHz ~ 928MHz Antenna Not Included, U.FL Surface Mount; PARTNO: 602-1889-ND
U5 = ruark2:VGDD79S433N0SA: -118dBm 433MHz 22dBm SPI SMD,11.5x11.5mm LoRa Modules ROHS; JLCPCB: C2976576
U6 = ruark2:V36SE12004NRFA: Isolated Module DC DC Converter 1 Output 12V 4.2A 18V - 75V Input; PARTNO: 941-1007-ND
U7 = ruark2:USBLC6-4SC6: 17V Clamp 5A (8/20µs) Ipp Tvs Diode Surface Mount SOT-23-6; PARTNO: 497-4492-1-ND
U8 = ruark2:ULN2003ADR: Bipolar (BJT) Transistor Array 7 NPN Darlington 50V 500mA Surface Mount 16-SOIC; PARTNO: 296-1368-1-ND
U9 = ruark2:UCC27517DBVR: Low-Side Gate Driver IC Inverting, Non-Inverting SOT-23-5, 4A, 8ns
U10 = ruark2:UCC27211: Half-Bridge Gate Driver IC Non-Inverting 8-SO PowerPad; PARTNO: 296-30344-1-ND
U11 = ruark2:TXEAADSANF-20.000000: 20MHz VCTCXO Clipped Sine Wave Oscillator 2.8 V ~ 3.3 V 4-SMD, No Lead; PARTNO: 1664-1240-1-ND
U12 = ruark2:TSC2046EQPWRQ1: Touch Screen Controllers 4-wire Touch Screen Controller; PARTNO: 2156-TSC2046EQPWRQ1-ND
U13 = ruark2:TSB572IST: General Purpose Amplifier 2 Circuit Rail-to-Rail 8-MiniSO; PARTNO: 497-16366-1-ND
U14 = ruark2:TS5A63157DBVR: MUX 1 Circuit IC Switch 2:1 10Ohm SOT-23-6; PARTNO: 296-21194-1-ND
U15 = ruark2:TS5A3160DBVR: MUX 1 Circuit IC Switch 2:1 900 mOhm SOT-23-6; PARTNO: 296-21189-1-ND
U16 = ruark2:TPS76133DBVR: Linear Voltage Regulator IC Positive Fixed 1 Output 100mA SOT-23-5; PARTNO: 296-11010-1-ND
U17 = ruark2:TPS63000DRCR: Buck-Boost Switching Regulator IC Positive Adjustable 1.2V 1 Output 1.6A (Switch) 10-VFDFN Exposed Pad; PARTNO: 296-19641-1-ND
U18 = ruark2:TPS62130AQRGTRQ1: Buck Switching Regulator IC Positive Adjustable 0.9V 1 Output 3A 16-VFQFN Exposed Pad; PARTNO: 296-40834-1-ND
U19 = ruark2:TPS61165DBVR: IC LED DRIVER RGLTR DIM SOT23-6; PARTNO: 296-27597-1-ND
U20 = ruark2:TPS61089RNRT: Boost Switching Regulator IC Positive Adjustable 4.5V 1 Output 7A 11-VFQFN; PARTNO: 296-46242-1-ND
U21 = ruark2:TPS61023DRLT: Boost Switching Regulator IC Positive Adjustable 2.2V 1 Output 3A SOT-563, SOT-666; PARTNO: 296-TPS61023DRLTCT-ND
U22 = ruark2:TPS54495: Buck Switching Regulator IC Positive Adjustable 0.76V 2 Output 4A, 2A 16-PowerTSSOP (0.173", 4.40mm Width); PARTNO: 296-30583-1-ND
U23 = ruark2:TPS25740B: USB, Type-C Controller PMIC 24-VQFN (4x4); PARTNO: 296-50077-1-ND
U24 = ruark2:TPS25740: USB, Type-C Controller PMIC 24-VQFN (4x4); PARTNO: 296-44487-1-ND
U25 = ruark2:TPS2553: Power Switch/Driver 1:1 N-Channel 1.5A SOT-23-6; PARTNO: 296-39380-1-ND
U26 = ruark2:TPS2513ADBVR: USB Dedicated Charging Port (DCP), Power Switch PMIC SOT-23-6
U27 = ruark2:TPS2065CDBVT: Power Switch/Driver 1:1 N-Channel 1A SOT-23-5; PARTNO: 296-29545-1-ND
U28 = ruark2:TPS2003CDRCR: Power Switch/Driver 1:2 N-Channel 2A 10-VSON (3x3) 2A; PARTNO: 296-40700-1-ND
U29 = ruark2:TPS7A1601AQDGNRQ1: Linear Voltage Regulator IC Positive Adjustable 60V 1 Output 100mA 8-HVSSOP
U30 = ruark2:TLV9061SQDBVRQ1: CMOS Amplifier 1 Circuit Rail-to-Rail SOT-23-6 10 MHz; PARTNO: 296-TLV9061SQDBVRQ1CT-ND
U31 = ruark2:TLV9002IDR: General Purpose Amplifier 2 Circuit Rail-to-Rail 8-SOIC 1MHz Rail to Rail; PARTNO: 296-47596-1-ND
U32 = ruark2:TLV320ADC3140: ADC, Audio 768k I²C, SPI 24-WQFN (4x4), 4-Channel, I2S/TDM; PARTNO: 296-TLV320ADC3140IRTWTCT-ND
U33 = ruark2:TLE83862ELXUMA1: IC REG CTRLR BOOST 14-SSOP; PARTNO: TLE83862ELXUMA1CT-ND
U34 = ruark2:TLC555CDG4: 555 Type, Timer/Oscillator (Single) IC 2.1MHz 8-SOIC; PARTNO: 296-52992-ND
U35 = ruark2:TC7660EOA: Charge Pump Switching Regulator IC Positive or Negative Fixed -Vin, 2Vin 1 Output 20mA 8-SOIC (0.154", 3.90mm Width); PARTNO: TC7660EOA-ND
U36 = ruark2:TC1071VCT713: Linear Voltage Regulator IC Positive Adjustable 1 Output 100mA SOT-23-5; PARTNO: TC1071VCT713CT-ND
U37 = ruark2:TA0419A: 441MHz Frequency General Purpose RF SAW Filter (Surface Acoustic Wave) 1.5dB 19MHz Bandwidth 8-SMD, No Lead; PARTNO: 4606-TA0419ACT-ND
U38 = ruark2:SX1276: IC RF TxRx Only 802.15.4 LoRa™ 137MHz ~ 1.02GHz 28-VQFN Exposed Pad; PARTNO: SX1276IMLTRTCT-ND
U39 = ruark2:SX1262S9S+T: -139dBm 915MHz 22dBm SPI SMD,16x16mm LoRa Modules ROHS
U40 = ruark2:SX1262IMLTRT: IC RF TxRx Only General ISM < 1GHz LoRaWAN 150MHz ~ 960MHz 24-VFQFN Exposed Pad; PARTNO: SX1262IMLTRTCT-ND
U41 = ruark2:STUSB4500QTR: USB Controller USB 2.0 I²C Interface 24-QFN (4x4); PARTNO: 497-18060-1-ND
U42 = ruark2:STM32F769BGT6: ARM® Cortex®-M7 series Microcontroller IC 32-Bit 216MHz 1MB (1M x 8) FLASH 208-LQFP (28x28); PARTNO: 497-16646-ND
U43 = ruark2:STM32F767ZIT6: ARM® Cortex®-M7 STM32F7 Microcontroller IC 32-Bit 216MHz 2MB (2M x 8) FLASH 144-LQFP (20x20); PARTNO: 497-16521-ND
U44 = ruark2:STM32F103C8T6TR: ARM® Cortex®-M3 STM32F1 Microcontroller IC 32-Bit 72MHz 64KB (64K x 8) FLASH 48-LQFP (7x7); PARTNO: 497-17666-1-ND
U45 = ruark2:STLVDS050: 2/2 Transceiver Full LVDS 16-SO; PARTNO: 497-2147-1-ND
U46 = ruark2:STG3157CTR: 1 Circuit IC Switch 2:1 15 Ohm SOT-323-6L; PARTNO: 497-2144-1-ND
U47 = ruark2:ST1480ABDR; PARTNO: 497-2046-1-ND
U48 = ruark2:ST1S40IPUR: Buck Switching Regulator IC Positive Adjustable 0.8V 1 Output 3A 8-VDFN Exposed Pad; PARTNO: 497-12084-1-ND
U49 = ruark2:SPAN02A-12: Isolated Module DC DC Converter 1 Output 12V 167mA 9V - 18V Input; PARTNO: 1866-4766-ND
U50 = ruark2:SN75179BD: 1/1 Transceiver Full RS422, RS485 8-SOIC 5V; PARTNO: 296-6860-5-ND
U51 = ruark2:SN74LVC138AQPWRQ1: Decoder/Demultiplexer 1 x 3:8 16-TSSOP; PARTNO: 296-28968-1-ND
U52 = ruark2:SN74LVC1G17DCKR: Buffer, Non-Inverting 1 Element 1 Bit per Element Push-Pull Output SC-70-5; JLCPCB: C10425; PARTNO: 296-11934-1-ND
U53 = ruark2:SN74LV4052APWR: Dual 4-Channel Analog Multiplexer; PARTNO: 296-3831-1-ND
U54 = ruark2:SN74LV4051ADR: 1 Circuit IC Switch 8:1 75Ohm 16-SOIC; PARTNO: 296-3827-1-ND
U55 = ruark2:SN74HCS00DR: NAND Gate IC 4 Channel Schmitt Trigger Input 14-SOIC; PARTNO: 296-SN74HCS00DRCT-ND
U56 = ruark2:SN74HC164DR: Shift Shift Register 1 Element 8 Bit 14-SOIC; PARTNO: 296-14838-1-ND
U57 = ruark2:SN65HVD231
U58 U59 = ruark2:SN65C1168ERGYR: 2/2 Transceiver Full RS422, RS485 16-VQFN (4x3.5); PARTNO: 296-21803-1-ND
U60 = ruark2:SKYA21003: IC RF SWITCH SPDT 6GHZ 12QFN; PARTNO: 863-1818-1-ND
U61 = ruark2:SKY13575-639LF: RF Switch IC 802.11a/b/g/n/ac SP4T 6GHz 50 Ohm 14-QFN (1.6x1.6); PARTNO: 863-1767-1-ND
U62 = ruark2:SKY13472: RF Switch IC SPDT 3GHz 50 Ohm 12-QFN (2x2); PARTNO: 863-1653-1-ND
U63 = ruark2:SKY13330-397LF: RF Switch IC W-CDMA SPDT 6GHz 50Ohm 12-QFN (2x2); PARTNO: 863-1643-1-ND
U64 = ruark2:SJ1-3523N: 3.50mm (0.141", 1/8", Mini Plug) - Headphone Phone Jack Stereo (3 Conductor, TRS) Connector Solder; PARTNO: CP1-3523N-ND
U65 = ruark2:SIC467ED-T1-GE3: Buck Switching Regulator IC Positive Adjustable 0.8V 1 Output 6A PowerPAK® MLP55-27 60V; PARTNO: SIC467ED-T1-GE3CT-ND
U66 = ruark2:SI8663BB-B-IU: General Purpose Digital Isolator 2500Vrms 6 Channel (3IN, 3OUT) 150Mbps 50kV/µs CMTI 16-SSOP (0.154", 3.90mm Width); PARTNO: 336-4304-ND
U67 = ruark2:SI4464: IC RF TxRx + MCU General ISM < 1GHz 119MHz ~ 1.05GHz 20-VFQFN Exposed Pad; PARTNO: 336-2472-5-ND
U68 = ruark2:SHT40-AD1B-R2: Temperature and Humidity Sensor ROHS; JLCPCB: C2909890
U69 = ruark2:RY8310: 30V 1.2A 1.4MHz PWM SYN Step-Down Regulator
U70 = ruark2:RP2040: Check availability; AVAILABILITY: Not in stock; DESCRIPTION: RP2040 chip for Raspberry Pi Pico - ARM® Cortex®-M0+ MCU 32-Bit; MF: Raspberry Pi; MP: RP2040; PACKAGE: None; PARTNO: 2648-SC0914(13)CT-ND; PRICE: None
U71 = ruark2:RFM98PW: 433 MHz 1W LoRa Module
U72 = ruark2:RFM-0505S: Isolated Module DC DC Converter 1 Output 5V 200mA - 5V Input; PARTNO: 945-3159-ND
U73 = ruark2:RASPBERRY_PICO: Raspberry Pi Pico
U74 = ruark2:PE42441C-Z: RF Switch IC WLAN SP4T 8GHz 50 Ohm 32-LGA (5x5); PARTNO: 1046-1108-1-ND
U75 = ruark2:PDSE1-S5-S9-S: Isolated Module DC DC Converter 1 Output 9V 111mA 4.5V - 5.5V Input; PARTNO: 102-6292-ND
U76 = ruark2:PDSE1-S5-S5-S: Isolated Module DC DC Converter 1 Output 5V 111mA 4.5V - 5.5V Input; PARTNO: 102-6291-ND
U77 = ruark2:PCM1681PWPR: DAC, Audio 24 b 192k DSP, I²S/PCM 28-HTSSOP, 8-CHANNEL; PARTNO: 296-41371-1-ND
U78 = ruark2:P78E05-1000: Non-Isolated PoL Module DC DC Converter 1 Output 5V 1A 8V - 36V Input; PARTNO: 102-5018-ND
U79 = ruark2:OPA2320AIDGKR: CMOS OPAMP OP-AMP 2 Circuit Rail-to-Rail 20MHz 8-VSSOP; PARTNO: 296-28067-1-ND
U80 = ruark2:OPA211AIDR: General Purpose Amplifier 1 Circuit Rail-to-Rail 8-SOIC Low Noise; PARTNO: 296-22634-1-ND
U81 = ruark2:NE555PSR: 555 Type, Timer/Oscillator (Single) IC 100kHz 8-SO; PARTNO: 296-6502-1-ND
U82 = ruark2:NCV5183DR2G: Half-Bridge Gate Driver IC Non-Inverting 8-SOIC 4.3A; PARTNO: NCV5183DR2GOSCT-ND
U83 = ruark2:NCP5901BDR2G: Internal Dead Time Half-Bridge Gate Driver IC 8-SOIC; PARTNO: NCP5901BDR2GOSCT-ND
